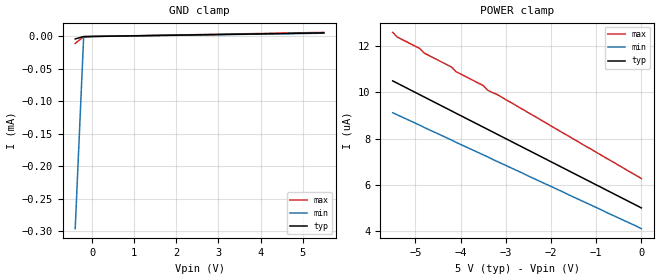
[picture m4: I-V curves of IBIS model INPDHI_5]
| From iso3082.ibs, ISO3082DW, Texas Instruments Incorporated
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|   Driver Enable 5V
[Model]   INPDHI_5
Model_type   Input
|Signals   DE
Vinh = 2.0
Vinl = 0.8
|   typ   min   max
C_comp   1.3pF   1.1pF   1.5pF
|   typ   min   max
[Temperature Range]   27   -40   85
[Voltage range]   5.0V   4.5V   5.5V
[GND_clamp]
|   Voltage   I(typ)   I(min)   I(max)
-400mV    -3.79uA    -296uA     -10.8uA
-200mV    -202nA     -1.2uA     -230nA
0V        0A         0A         0A
5.5V      5.5uA      5.02uA     6.27uA
[Power_clamp]
| Note that the[POWER_clamp]voltage table is referenced to Vcc
| and is calculated using Vtable=Vcc - Vmeasured.
|   Voltage   I(typ)   I(min)   I(max)
-5.5V     10.5uA     9.12uA     12.6uA
-5.4V     10.4uA     9.03uA     12.4uA
-4.9V     9.9uA      8.58uA     11.9uA
-4.8V     9.8uA      8.48uA     11.7uA
-4.2V     9.2uA      7.94uA     11.1uA
-4.1V     9.1uA      7.84uA     10.9uA
-3.5V     8.5uA      7.3uA      10.3uA
-3.4V     8.4uA      7.21uA     10.1uA
-3.1V     8.1uA      6.93uA     9.81uA
0V        5uA        4.1uA      6.27uA
